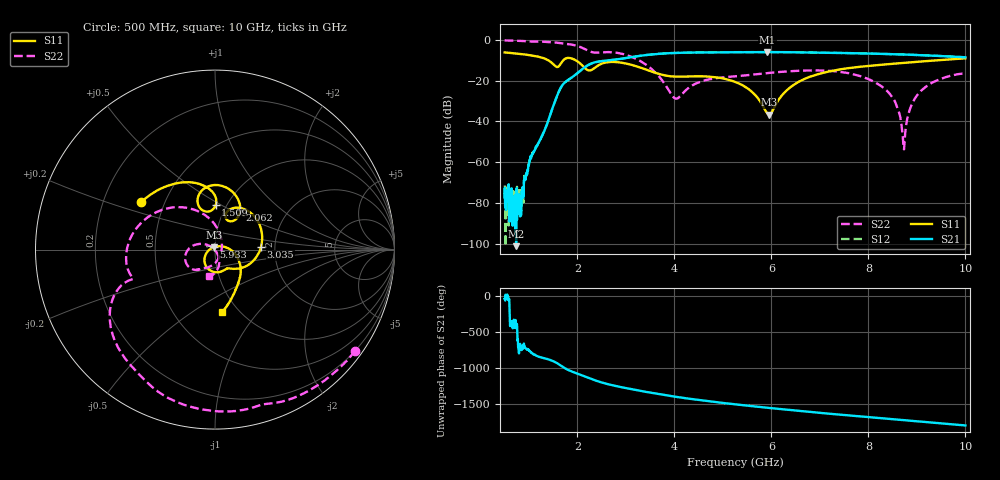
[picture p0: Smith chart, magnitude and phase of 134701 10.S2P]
!  2-Port S-parameters saved by WinCal
! VAR MeasName=S-Parameters (CALIBRATED_DATA) read from VNA (N5242A)
! VAR MeasDate=2013-7-3 16:28:40
! VAR NAME=134701 10
! VAR FILENAME=134701 10.S2P
! VAR DATE=2013-7-3 16:28:40
! VAR PHYS_PORTS=1,2
# Hz S MA R 50
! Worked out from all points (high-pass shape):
!   1601 points, 500 MHz to 10 GHz, reference 50 ohm
!   highest |S21| = -6.03 dB at 5.915 GHz (marker M1); lowest = -101.2 dB at 737.5 MHz (marker M2)
!   |S21| within 3 dB of the highest: 2.975 GHz to end of sweep
!   lowest |S11| = -36.8 dB at 5.951 GHz (marker M3), VSWR 1.03, Z = 49.5 + j1.36 ohm
!   |S11| at or under -10 dB: 1.397 GHz to 1.712 GHz (314.4 MHz wide, 20.2 % of centre); 1.963 GHz to 9.454 GHz (7.491 GHz wide, 131 % of centre)
!   |S22| runs from -53.7 to -0.3 dB; largest |S21 - S12| = 0.0028
!   S11 on the Smith chart (normalised r, x): 500 MHz: 0.37, +0.25; 1.509 GHz: 0.89, +0.47; 2.062 GHz: 1.18, +0.56; 3.035 GHz: 1.69, +0.06; 5.933 GHz: 0.98, +0.03; 10 GHz: 0.84, -0.67
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5e8  0.4913 147.6  0.0001365 -41.0  0.0001432 -31.0  0.9629 -35.9
7.375e8  0.4606 134.3  8.755e-06 -88.4  0.0001565 -13.5  0.9478 -52.8
8.44375e8  0.4464 128.2  0.0001189 -35.3  6.367e-05 74.1  0.9377 -60.4
1.028438e9  0.4188 116.9  0.001203 -53.4  0.001253 -58.3  0.9026 -72.8
1.509375e9  0.2478 89.1  0.02498 168.6  0.02492 168.2  0.8666 -107.7
2.061562e9  0.2607 57.4  0.1748 -16.1  0.1746 -16.1  0.6642 -151.3
2.085312e9  0.2454 55.8  0.1844 -22.2  0.1839 -22.2  0.6462 -153.0
2.435625e9  0.2376 69.9  0.2926 -110.1  0.2919 -110.1  0.485 -161.2
3.035312e9  0.2573 3.5  0.3628 153.6  0.3624 153.7  0.4144 154.0
3.670625e9  0.1474 -46.8  0.4532 75.5  0.4531 75.5  0.1311 87.6
4.03875e9  0.1251 -58.5  0.4767 36.2  0.4767 36.2  0.03618 -12.1
5.25e9  0.09278 -128.4  0.4973 -66.8  0.4976 -66.8  0.1272 -124.6
5.915e9  0.01577 132.8  0.4997 -114.2  0.4987 -114.3  0.1525 -132.0
5.932812e9  0.01507 121.4  0.4991 -115.5  0.4985 -115.5  0.1534 -132.3
5.950625e9  0.01451 109.4  0.4991 -116.7  0.4983 -116.8  0.1541 -132.5
6.835312e9  0.1288 -17.9  0.4899 -175.0  0.4898 -175.0  0.1773 -152.4
8.420625e9  0.253 -63.3  0.4466 89.5  0.4469 89.5  0.05067 148.9
8.59875e9  0.2636 -65.8  0.4407 79.2  0.4411 79.3  0.02152 143.6
8.735312e9  0.2713 -67.9  0.4345 71.2  0.4362 71.3  0.002066 -122.8
8.871875e9  0.2799 -69.8  0.4281 63.5  0.4299 63.4  0.02234 -61.8
9.079688e9  0.2931 -72.5  0.4192 51.6  0.4204 51.5  0.05528 -66.9
1e10  0.3515 -83.5  0.3722 0.0  0.3735 -0.0  0.1522 -101.6
